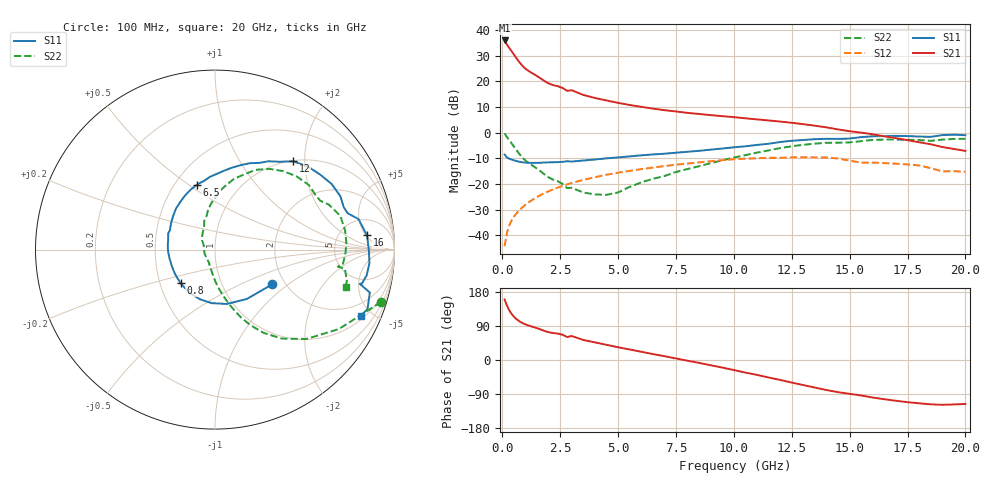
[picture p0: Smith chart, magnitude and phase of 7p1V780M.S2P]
! Infineon Technologies  Discrete & RF Semiconductors
! bfp620
! VCE =  1.7 V,  IC =  80 mA
! Common Emitter S-Parameters:  Sep 2002
# GHz  S  MA  R  50
!  f  S11  S21  S12  S22
! GHz  MAG  ANG  MAG  ANG  MAG  ANG  MAG  ANG
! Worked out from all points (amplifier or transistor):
!   59 points, 100 MHz to 20 GHz, reference 50 ohm
!   highest |S21| = 36.0 dB at 100 MHz (marker M1)
!   |S21| within 3 dB of that: start of sweep to 306.7 MHz
!   unconditionally stable (mu >= 1): 1.955 GHz to 2.33 GHz; 3.038 GHz to 9.952 GHz; 17.15 GHz to end of sweep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
!   at 1 GHz: K = 0.90, MSG = 26.6 dB, |S12| = -28.1 dB
!   at 5.5 GHz: K = 1.04, MAG = 11.6 dB, |S12| = -14.9 dB
!   at 20 GHz: K = 1.28, MAG = 0.9 dB, |S12| = -15.3 dB
!   S11 on the Smith chart (normalised r, x): 100 MHz: 1.72, -0.77; 800 MHz: 0.64, -0.25; 6.5 GHz: 0.64, +0.54; 12 GHz: 1.01, +1.75; 16 GHz: 9, +5; 20 GHz: 1.20, -4.33
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0.1  0.3736 -31.1  62.95 159.7  0.0061 78.7  0.9706 -17.5
0.2  0.3274 -57.1  52.37 143.8  0.0111 73.9  0.8199 -32.7
0.3  0.3099 -77.7  45.01 131.3  0.0155 71.5  0.7118 -44.4
0.4  0.2989 -93.8  38.92 121.7  0.0193 70.0  0.6198 -53.1
0.5  0.2889 -107.1  33.56 114.4  0.0229 68.9  0.5374 -59.7
0.6  0.2799 -118.3  28.91 108.5  0.0262 68.2  0.4649 -64.9
0.7  0.2726 -127.9  25.02 103.8  0.0295 67.6  0.4038 -69.1
0.8  0.2672 -136.0  21.91 99.8  0.0327 67.2  0.3545 -72.4
0.9  0.2633 -142.7  19.53 96.6  0.0359 66.8  0.3159 -75.2
1.1  0.2588 -153.0  16.38 91.7  0.0424 66.1  0.2635 -79.6
1.9  0.2623 179.7  9.66 75.2  0.0686 60.9  0.1441 -94.4
2.8  0.2764 160.5  6.556 60.6  0.0978 53.3  0.0832 -113.5
3  0.2735 157.2  6.718 63.3  0.1042 51.5  0.084 -112.0
3.5  0.2861 148.7  5.437 52.8  0.1201 46.7  0.068 -130.0
6.5  0.3758 105.4  2.946 15.7  0.2081 17.1  0.1256 121.4
7  0.3881 99.1  2.749 10.1  0.2226 12.2  0.1426 115.2
10.5  0.5422 63.0  1.906 -33.2  0.3107 -27.7  0.364 80.3
12  0.6563 48.6  1.645 -52.6  0.3228 -45.4  0.4996 62.9
13.5  0.7456 29.3  1.367 -72.7  0.3287 -64.1  0.6106 42.0
16  0.8504 5.4  0.929 -99.1  0.2605 -87.9  0.723 15.1
17  0.8638 -4.9  0.784 -107.6  0.2478 -95.9  0.7329 3.0
20  0.8927 -24.3  0.441 -116.0  0.1726 -105.6  0.7576 -15.9
